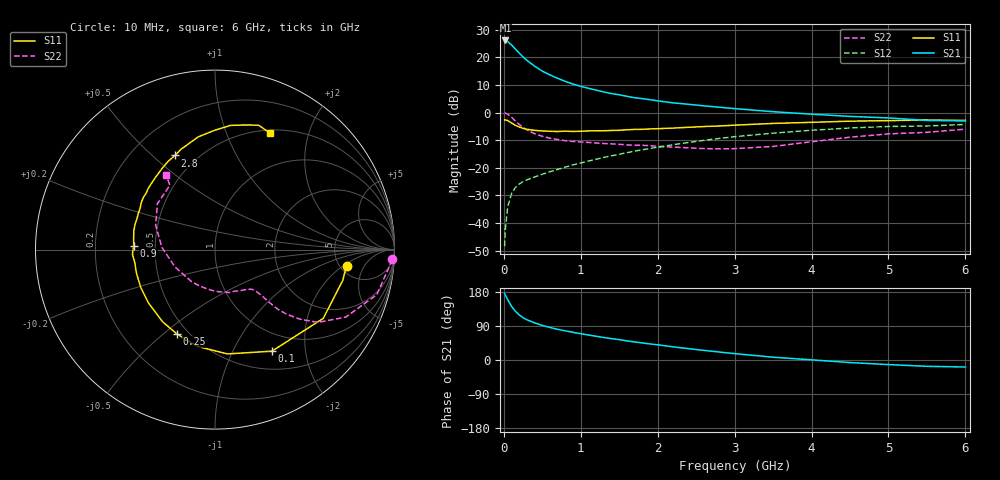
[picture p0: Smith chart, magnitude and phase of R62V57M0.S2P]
! SIEMENS Small Signal Semiconductors
! BFR193
! Si NPN RF Bipolar Junction Transistor in SOT23
! VCE = 2.5 V  IC = 7 mA
! Common Emitter S-Parameters:  May  1996
# GHz  S  MA  R  50
!  f  S11  S21  S12  S22
! GHz  MAG  ANG  MAG  ANG  MAG  ANG  MAG  ANG
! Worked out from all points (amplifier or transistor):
!   36 points, 10 MHz to 6 GHz, reference 50 ohm
!   highest |S21| = 26.1 dB at 20 MHz (marker M1)
!   |S21| within 3 dB of that: start of sweep to 145.9 MHz
!   unconditionally stable (mu >= 1): 815.2 MHz to 2.028 GHz
!   at 250 MHz: K = 0.53, MSG = 22.6 dB, |S12| = -25.0 dB
!   at 1.4 GHz: K = 1.05, MAG = 9.9 dB, |S12| = -15.7 dB
!   at 6 GHz: K = 0.96, MSG = 0.6 dB, |S12| = -4.3 dB
!   lowest NFmin = 1.20 dB at 450 MHz
!   S11 on the Smith chart (normalised r, x): 10 MHz: 5.74, -2.24; 100 MHz: 0.74, -1.44; 250 MHz: 0.43, -0.55; 900 MHz: 0.38, +0.02; 2.8 GHz: 0.38, +0.59; 6 GHz: 0.53, +1.43
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0.01  0.738 -6.9  20.1 175.8  0.0038 87.5  0.9877 -3.2
0.02  0.7323 -13.5  20.18 171.1  0.0079 85.3  0.9712 -6.4
0.05  0.7146 -32.4  19.19 159.2  0.0195 75.2  0.9356 -15.6
0.1  0.6488 -60.7  16.75 141.9  0.034 63.7  0.8198 -27.3
0.15  0.5855 -83.1  14.09 128.4  0.0439 56.8  0.7019 -35.3
0.2  0.5484 -100.2  11.9 119.1  0.0506 53.3  0.6097 -39.4
0.25  0.5153 -114.4  10.15 111.6  0.0561 51.2  0.5379 -42.0
0.3  0.4969 -125.9  8.81 106.0  0.0604 51.2  0.4833 -43.5
0.4  0.4749 -141.5  6.912 98.0  0.0682 51.8  0.4143 -44.3
0.5  0.4644 -152.9  5.627 91.3  0.0763 52.9  0.3703 -44.5
0.6  0.4569 -163.2  4.793 85.8  0.0848 54.7  0.3422 -45.0
0.7  0.4527 -170.7  4.159 80.9  0.0934 56.4  0.3236 -45.5
0.9  0.4534 177.4  3.267 73.0  0.1128 58.6  0.2991 -47.4
1.1  0.464 167.1  2.746 65.9  0.1322 59.6  0.2871 -50.8
1.3  0.4679 158.3  2.356 59.4  0.1536 59.8  0.2744 -54.9
1.6  0.4874 147.4  1.965 50.5  0.1876 59.4  0.2595 -62.9
2.2  0.5222 129.2  1.497 34.7  0.2612 55.1  0.2368 -83.7
2.8  0.5701 113.0  1.248 21.1  0.3391 48.1  0.2199 -114.1
3.5  0.6348 98.5  1.035 7.4  0.4233 37.4  0.2433 -156.7
4.5  0.6972 82.9  0.851 -6.8  0.525 21.6  0.3574 157.8
5.5  0.7346 70.7  0.719 -16.7  0.5709 5.4  0.4381 125.0
6  0.7186 65.0  0.706 -18.4  0.6085 0.7  0.5 123.2
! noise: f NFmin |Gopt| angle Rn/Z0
0.45  1.2  0.24  125  0.12
0.9  1.25  0.36  154  0.11
1.8  2  0.55  -156  0.13
